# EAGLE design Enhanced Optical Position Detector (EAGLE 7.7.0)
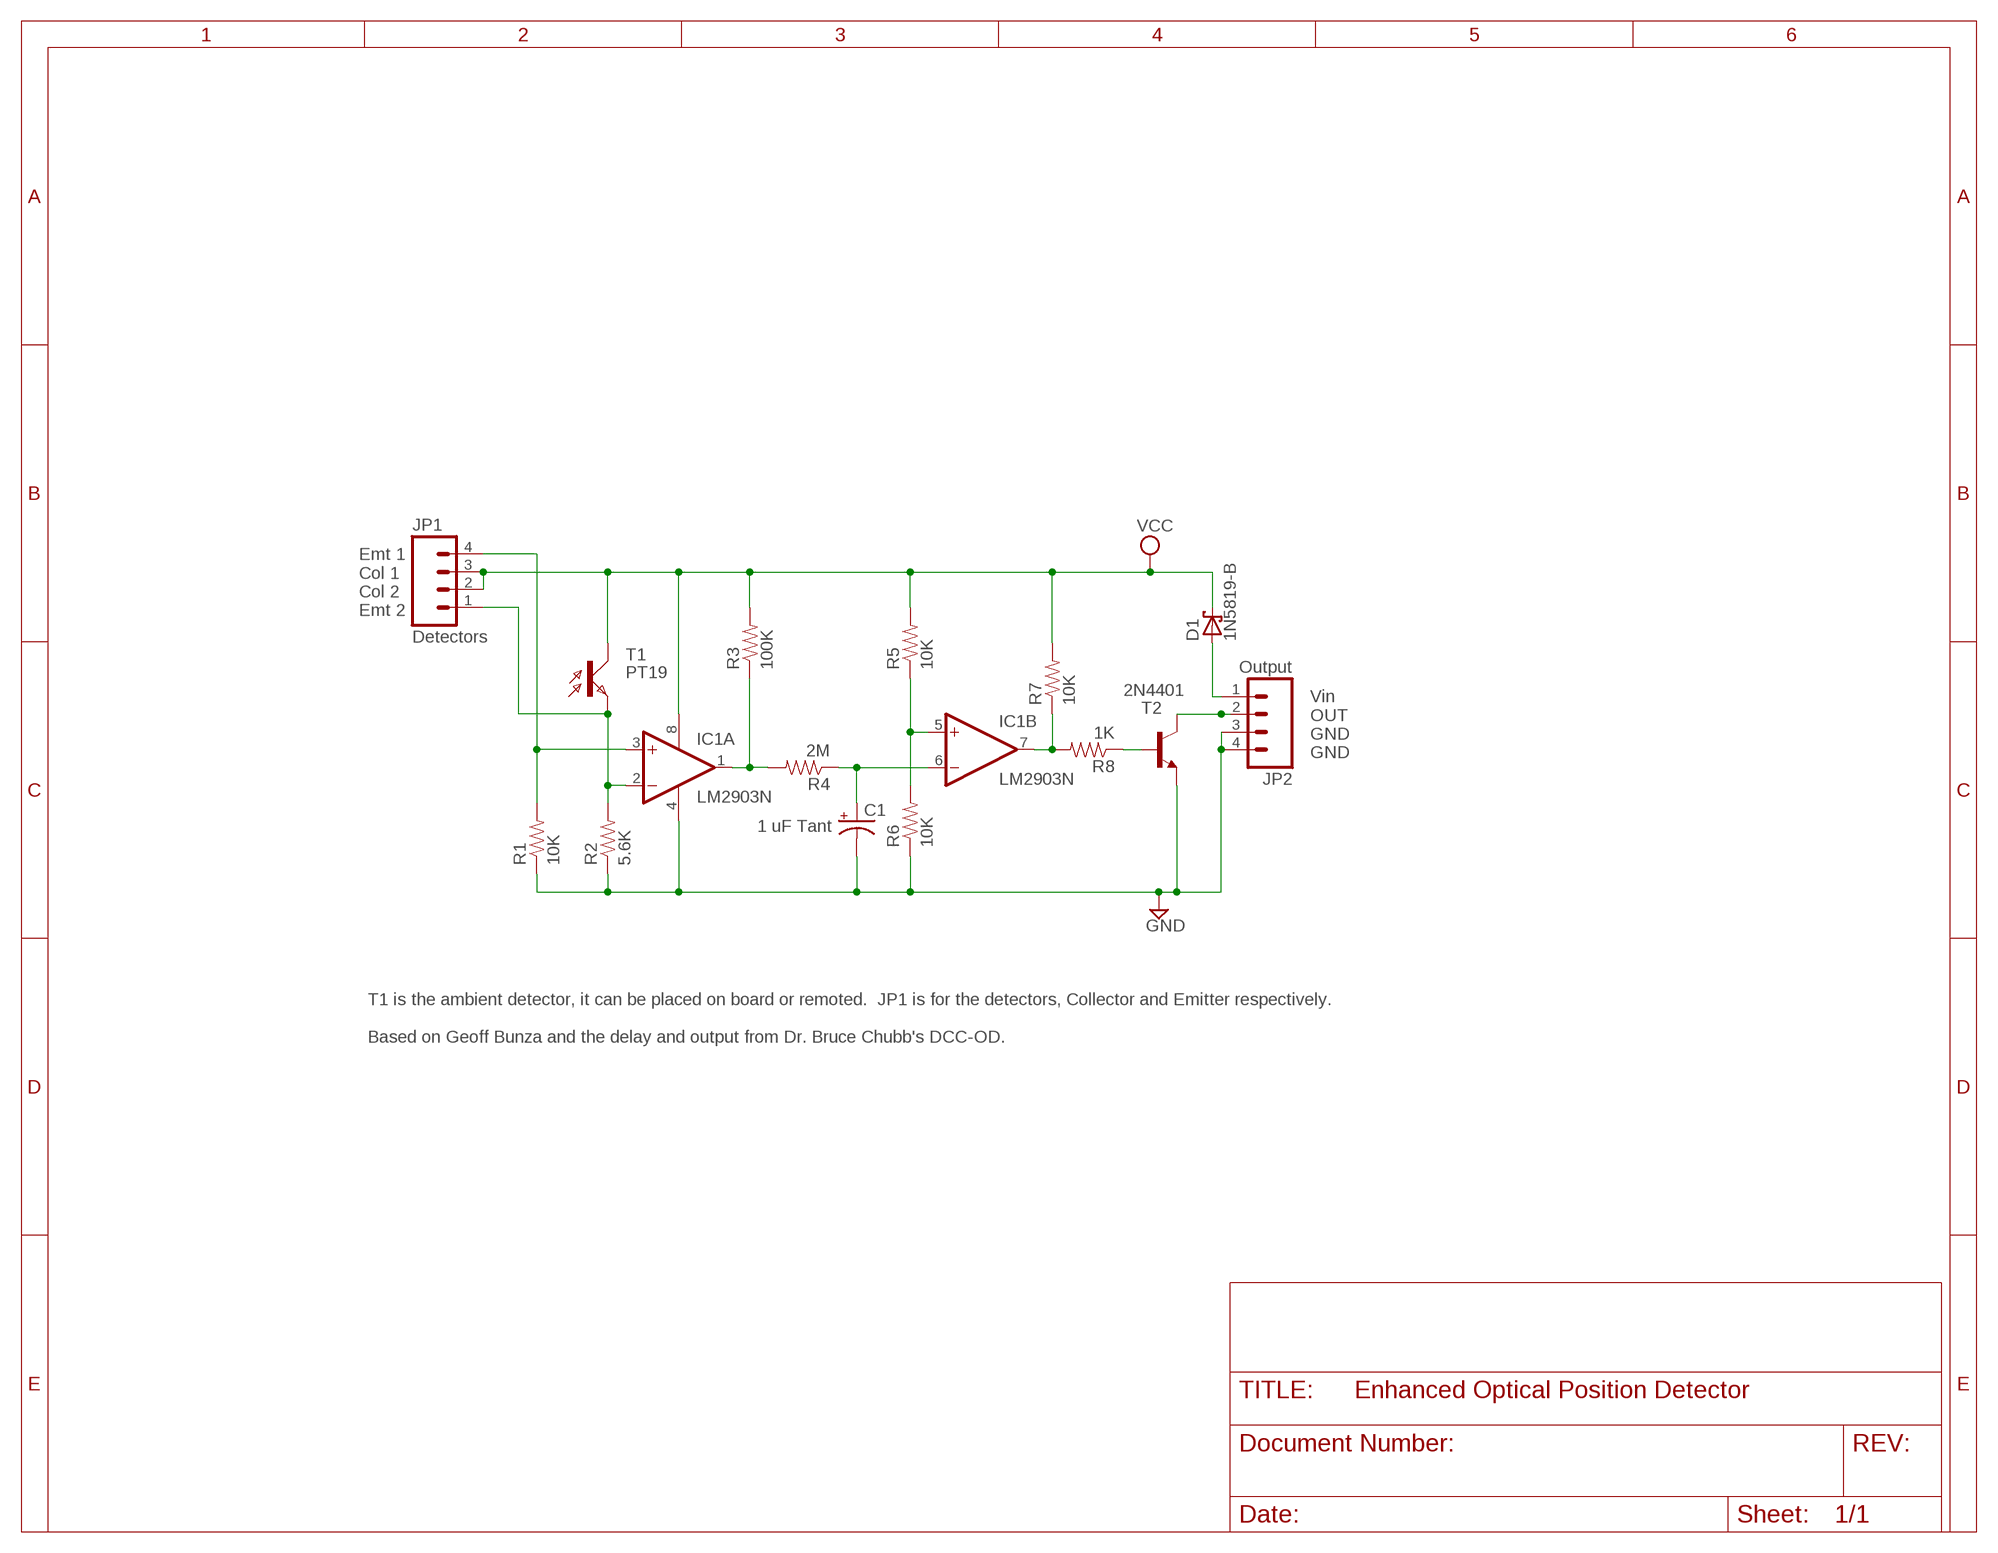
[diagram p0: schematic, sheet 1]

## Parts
C1  1 uF Tant  CPOL-USE2.5-5  [E2,5-5]
D1  1N5819-B  [DO41-7.6]
IC1  LM2903N  [DIL08]
JP1  Detectors  M04LOCK  [1X04_LOCK]
JP2  Output  M04LOCK  [1X04_LOCK]
R1  10K  RESISTORPTH-1/4W  [AXIAL-0.4]
R2  5.6K  RESISTORPTH-1/4W  [AXIAL-0.4]
R3  100K  RESISTORPTH-1/4W  [AXIAL-0.4]
R4  2M  RESISTORPTH-1/4W  [AXIAL-0.4]
R5  10K  RESISTORPTH-1/4W  [AXIAL-0.4]
R6  10K  RESISTORPTH-1/4W  [AXIAL-0.4]
R7  10K  RESISTORPTH-1/4W  [AXIAL-0.4]
R8  1K  RESISTORPTH-1/4W  [AXIAL-0.4]
T1  PT19  BPX81  [BPX81]
T2  2N4401  2N3904-NPN-TO92-EBC  [TO92-EBC]

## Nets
GND: C1.- IC1.4(P:V-) JP2.3 JP2.4 R1.P$1 R2.P$1 R6.P$1 T2.E
N$1: IC1.2(A:-IN) JP1.1 R2.P$2 T1.E
N$2: C1.+ IC1.6(B:-IN) R4.P$1
N$3: IC1.3(A:+IN) JP1.4 R1.P$2
N$4: IC1.1(A:OUT) R3.P$1 R4.P$2
N$5: IC1.7(B:OUT) R7.P$1 R8.P$2
N$6: IC1.5(B:+IN) R5.P$1 R6.P$2
N$7: R8.P$1 T2.B
N$8: JP2.2 T2.C
VCC: D1.C IC1.8(P:V+) JP1.2 JP1.3 R3.P$2 R5.P$2 R7.P$2 T1.C
VIN: D1.A JP2.1

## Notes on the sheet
- Emt 1
  Col 1
  Col 2
  Emt 2
- Vin
  OUT
  GND
  GND
- T1 is the ambient detector, it can be placed on board or remoted.  JP1 is for the detectors, Collector and Emitter respectively.
  
  Based on Geoff Bunza and the delay and output from Dr. Bruce Chubb's DCC-OD.

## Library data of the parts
C1 = rcl:CPOL-US: POLARIZED CAPACITOR, American symbol
D1 = diode:1N581*: 1.0A SCHOTTKY BARRIER RECTIFIER
IC1 = linear:LM2903: COMPARATOR
JP1 JP2 = SparkFun-Connectors:M04: Header 4 Standard 4-pin 0.1" header. Use with straight break away headers (SKU : PRT-00116), right angle break away headers (PRT-00553), swiss pins (PRT-00743), machine pins (PRT-00117), and female headers (PRT-00115). Molex polarized connector foot print use with SKU : PRT-08231 with associated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
R1-R8 = SparkFun-Resistors:RESISTOR: Resistor
T1 = opto-trans-siemens:BPX81: PHOTO TRANSISTOR; OC_FARNELL: unknown; OC_NEWARK: unknown
T2 = transistor-neu-to92:*-NPN-: NPN Transistror

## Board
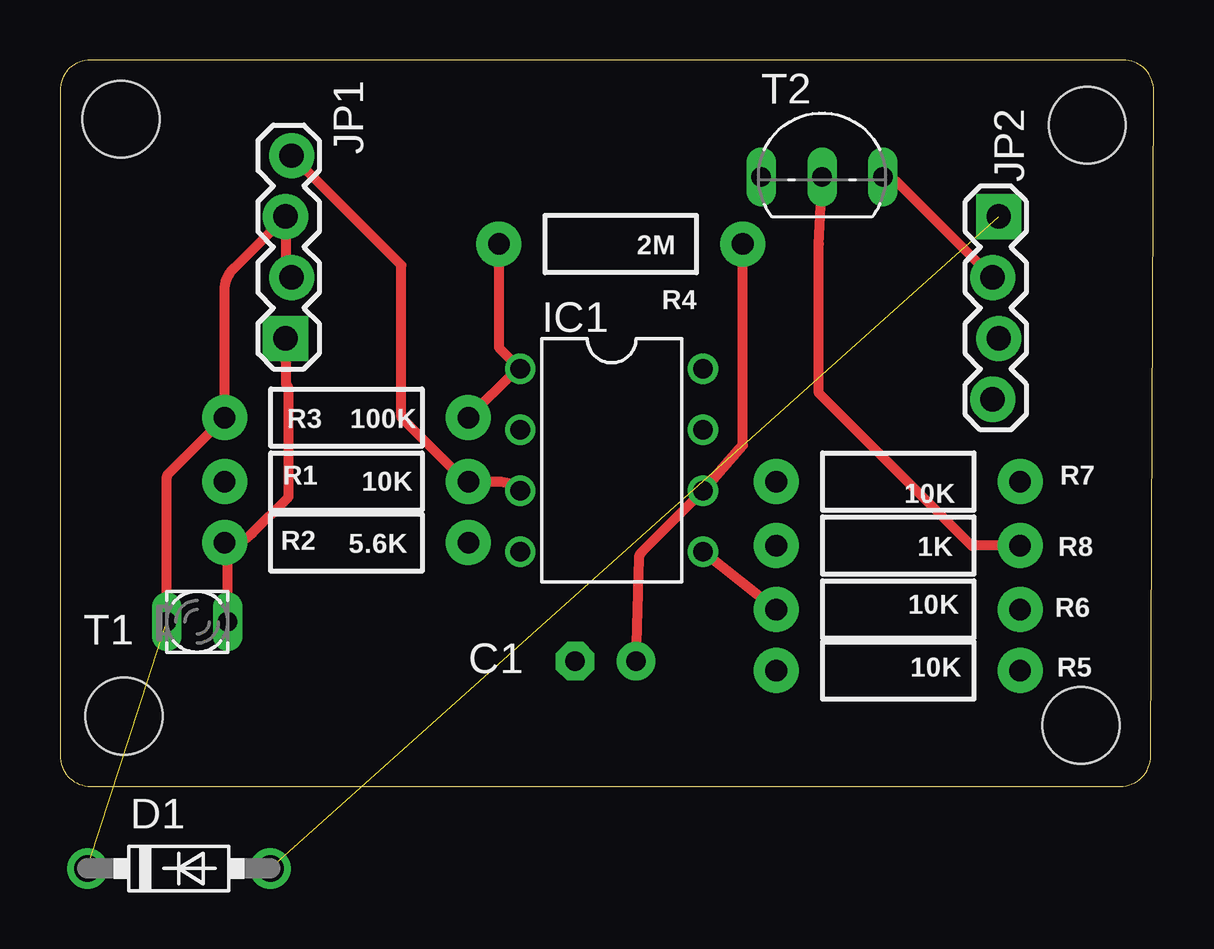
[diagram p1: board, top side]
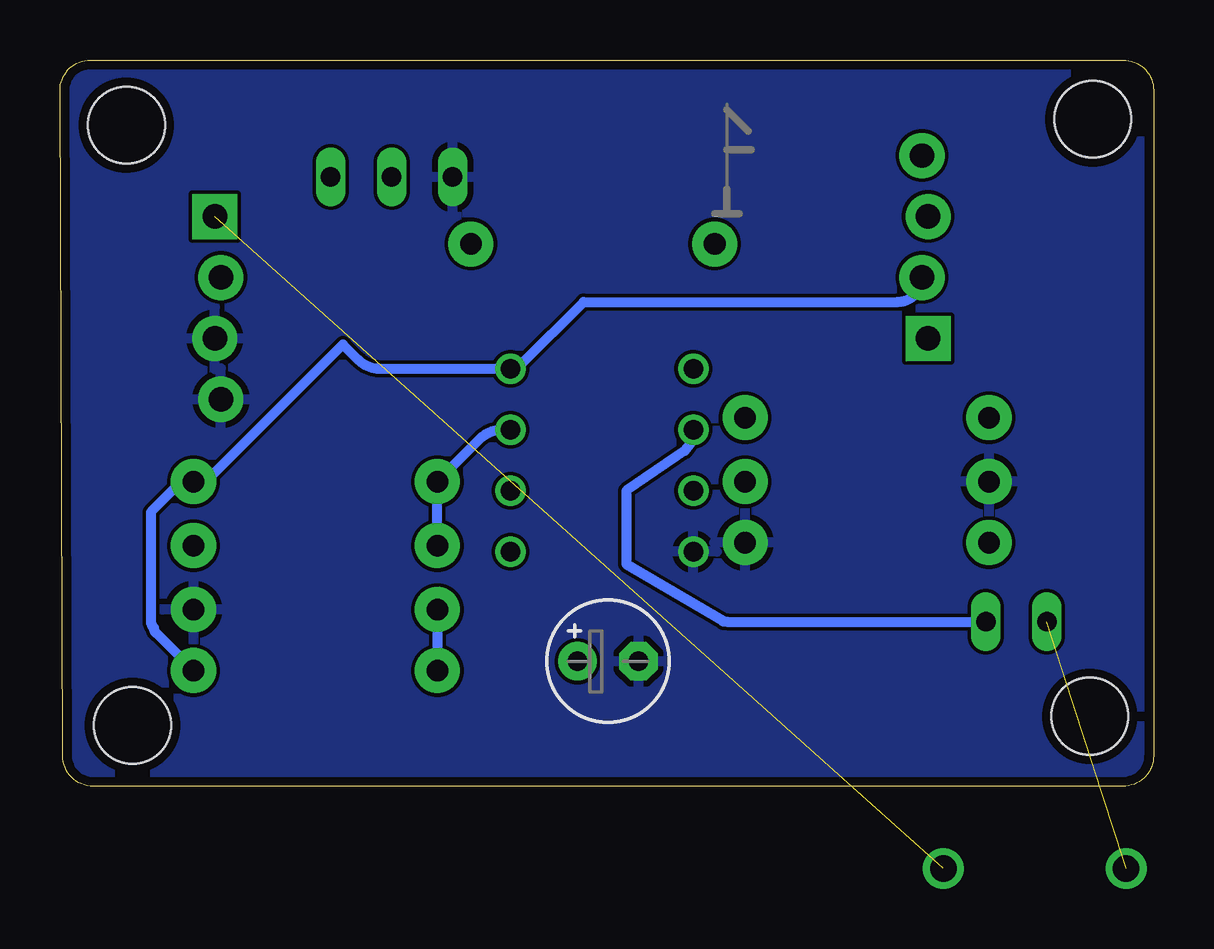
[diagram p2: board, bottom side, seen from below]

Size 45.57 x 30.28 mm. Coordinates in mm from the lower left corner, seen from the top.
Outline: 0,29.01 0,1.27 arc90 1.27,0 44.18,0 arc90 45.45,1.27 45.57,29 arc90 44.3,30.28 1.27,30.28 arc90 0,29.01
Copper layers (1*16): Top 0.0356mm / dielectric 1.5011mm / Bottom 0.0356mm
Design rules "LaenPCBOrder": minimum track width 6mil, minimum drill 13mil, track to track 6mil, track to pad 6mil, pad to pad 6mil, via to via 6mil, smd to smd 6mil, copper to edge 15mil, drill to drill 6mil, minimum pad ring 7mil, minimum via ring 7mil, stop-mask expansion 4mil, vias tented up to drill 0mil, thermal gap 10mil
Holes 3.2 mm at 2.54,27.81 42.8,27.56 2.67,2.92 42.54,2.54

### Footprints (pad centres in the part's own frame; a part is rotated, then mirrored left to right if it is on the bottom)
E2,5-5 = drill 0.813 pad 1.6: + -1.27,0 | drill 0.813 pad 1.6 octagon: - 1.27,0
DO41-7.6 = drill 1.1 pad 1.7: A 3.81,0; C -3.81,0
DIL08 = drill 0.813 pad 1.27: 1 -3.81,-3.81; 2 -1.27,-3.81; 3 1.27,-3.81; 4 3.81,-3.81; 5 3.81,3.81; 6 1.27,3.81; 7 -1.27,3.81; 8 -3.81,3.81
1X04_LOCK = drill 1.016 pad 1.88 square: 1 0,0.127 | drill 1.016 pad 1.88: 2 2.54,-0.127; 3 5.08,0.127; 4 7.62,-0.127
AXIAL-0.4 = drill 0.9 pad 1.88: P$1 -5.08,0; P$2 5.08,0
BPX81 = drill 0.813 long: C 1.27,0; E -1.27,0
TO92-EBC = drill 0.813 long: B 0,-1.27; C 2.54,-1.27; E -2.54,-1.27

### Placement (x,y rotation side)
C1  22.73,5.21 0 bottom
D1  not placed on the board
IC1  22.99,13.59 270 top
JP1  9.52,18.67 90 top
JP2  38.99,23.75 270 top
R1  11.94,12.7 0 top
R2  11.94,10.16 180 top
R3  11.94,15.37 180 top
R4  23.37,22.61 180 top
R5  34.92,4.83 0 top
R6  34.92,7.37 180 top
R7  34.92,12.7 0 top
R8  34.92,10.03 180 top
T1  5.71,6.86 180 top
T2  31.75,26.67 0 top
U$1  [MRCSLOGOBTM]  11.43,23.37 0 top
U$3  [CA-PROP65WARNING]  23.11,18.54 90 top

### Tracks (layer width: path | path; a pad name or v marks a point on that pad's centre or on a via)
GND
  pour Bottom: 0.38,29.97 45.21,29.97 44.96,0.51 0.51,0.51
N$1
  Top 0.406: T1.E 6.99,9.91 R2.P$2 7.09,10.16 arc45 7.99,10.53 9.52,12.06 9.52,16.51 arc45 9.43,16.73 JP1.1
  Bottom 0.406: IC1.2 arc45 19.54,13.99 21.97,12.32 21.97,9.25 17.96,6.89 arc-45 17.78,6.86 T1.E
N$2
  Top 0.406: R4.P$1 28.45,14.22 IC1.6 24.22,9.74 arc45 24.13,9.52 C1.+
N$3
  Top 0.406: IC1.3 IC1.3 arc45 18.27,12.7 R1.P$2 arc-45 16.8,12.79 14.22,15.37 14.22,21.72 JP1.4
N$4
  Top 0.406: R4.P$2 18.29,18.29 IC1.1 arc45 18.96,17.31 R3.P$1
N$5
  Bottom 0.406: R8.P$2 R7.P$1 28.06,14.49 arc45 27.16,14.86 IC1.7
N$6
  Top 0.406: IC1.5 R6.P$2
  Bottom 0.406: R6.P$2 R5.P$1
N$7
  Top 0.406: R8.P$1 37.97,10.03 31.62,16.38 31.62,22.61 T2.B
N$8
  Top 0.406: T2.C arc-45 34.94,25.13 JP2.2
VCC  (1 unrouted)
  Top 0.406: T1.C 4.45,12.83 arc-45 4.54,13.04 R3.P$2 6.86,20.68 arc-45 7.23,21.58 JP1.3 9.4,21.82 arc45 JP1.2
  Bottom 0.406: R5.P$2 41.57,6.39 arc45 41.66,6.6 arc45 41.78,6.91 41.78,11.43 40.87,12.34 arc45 R7.P$2 arc-45 39.14,13.06 33.78,18.41 33.14,17.77 arc-45 32.24,17.4 IC1.8 arc-45 26.36,17.58 23.75,20.19 10.67,20.19 arc-90 JP1.2
VIN  (1 unrouted)

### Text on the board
tDocu: E1 / C1 / C2 / E2 | VCC / OUT / GND / GND | DAPD-DFM Geoff Bunza 2015, Seth Neumann 2017
bDocu: MRCS DAPD-DFM / Based on Geoff Bunza 2015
